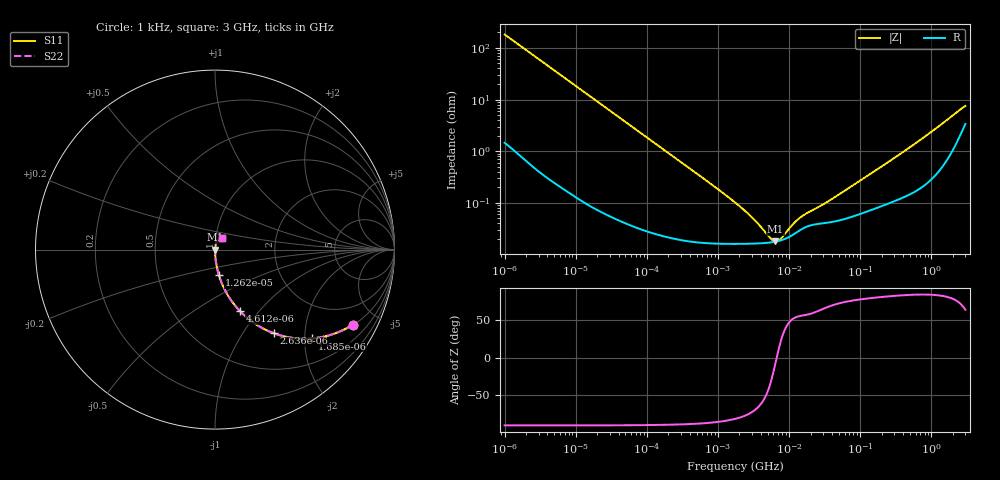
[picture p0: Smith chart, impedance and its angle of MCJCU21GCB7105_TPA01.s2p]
! MCJCU21GCB7105_TPA01  S-PARAMETER MODEL  ( Standard Model )
! Model Generated by TAIYO YUDEN Corporation (http://www.ty-top.com)
! Version 1.0
! TAIYO YUDEN Control No. 220601
! Copyright(c) 2015 TAIYO YUDEN CO.,LTD. All Rights Reserved.
! Product Description (link to TY-COMPAS)
! https://ds.yuden.co.jp/TYCOMPAS/or/detail?pn=MCJCU21GCB7105KTPA01&u=M
! Products Name : Multilayer Ceramic Capacitors
! Characteristics :
!  Capacitance : 1 [uF] , Rated Voltage : 50 [V] , TCC : X7R
!  Case Size : 2.0 x 1.25 / 0.079 x 0.049 [mm/inch] , Thickness : 1.25 / 0.049 [mm/inch]
!  (Conditions: Temperature = 25 [degC] , DC Bias Voltage = 0 [V])
! External Node Assignments :
!  1  o---| |---o  2
! GND o---------o GND
! Frequency Range : 1kHz  -  3GHz  [ 401 STEP ]
# MHZ S RI R 50
! Freq[MHz].  S11 Real  S11 Imag  S21 Real  S21 Imag  S12 Real  S12 Imag  S22 Real  S22 Imag
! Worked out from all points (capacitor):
!   401 points, 1 kHz to 3 GHz, reference 50 ohm
!   read as one part in series: C = 872 nF near 1.077 kHz
!   lowest |Z| = 17.9 mohm at 6.387 MHz (marker M1)
!   series resonance near 6.679 MHz, so ESL is about 650 pH
!   S11 on the Smith chart (normalised r, x): 1 kHz: 1.03, -3.64; 1.685 kHz: 1.02, -2.17; 2.636 kHz: 1.01, -1.39; 4.612 kHz: 1.01, -0.80; 12.62 kHz: 1.00, -0.29; 3 GHz: 1.07, +0.13
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0.001  0.7666 -0.419  0.2334 0.419  0.2334 0.419  0.7666 -0.419
0.001685  0.54 -0.4947  0.46 0.4947  0.46 0.4947  0.54 -0.4947
0.002636  0.3264 -0.4655  0.6736 0.4655  0.6736 0.4655  0.3264 -0.4655
0.004612  0.1382 -0.3418  0.8618 0.3418  0.8618 0.3418  0.1382 -0.3418
0.007215  0.0623 -0.2384  0.9377 0.2384  0.9377 0.2384  0.0623 -0.2384
0.01216  0.0234 -0.1477  0.9766 0.1477  0.9766 0.1477  0.0234 -0.1477
0.012621  0.0218 -0.1425  0.9782 0.1425  0.9782 0.1425  0.0218 -0.1425
0.03454  0.00335 -0.0533  0.9966 0.0533  0.9966 0.0533  0.00335 -0.0533
0.147855  0.000396 -0.0126  0.9996 0.0126  0.9996 0.0126  0.000396 -0.0126
1.732051  0.000162 -0.00101  0.9998 0.00101  0.9998 0.00101  0.000162 -0.00101
3.14518  0.000163 -0.000464  0.9998 0.000464  0.9998 0.000464  0.000163 -0.000464
5.502215  0.000172 -0.00011  0.9998 0.00011  0.9998 0.00011  0.000172 -0.00011
6.387174  0.000177 -2.53e-05  0.9998 2.53e-05  0.9998 2.53e-05  0.000177 -2.53e-05
7.696136  0.000189 8.05e-05  0.9998 -8.05e-05  0.9998 -8.05e-05  0.000189 8.05e-05
10.76485  0.000232 0.000274  0.9998 -0.000274  0.9998 -0.000274  0.000232 0.000274
13.46371  0.000283 0.000397  0.9997 -0.000397  0.9997 -0.000397  0.000283 0.000397
21.06097  0.000374 0.000613  0.9996 -0.000613  0.9996 -0.000613  0.000374 0.000613
39.69685  0.000427 0.0011  0.9996 -0.0011  0.9996 -0.0011  0.000427 0.0011
256.0921  0.00102 0.00629  0.999 -0.00629  0.999 -0.00629  0.00102 0.00629
1533.384  0.00706 0.0363  0.9929 -0.0363  0.9929 -0.0363  0.00706 0.0363
2489.759  0.0223 0.0577  0.9777 -0.0577  0.9777 -0.0577  0.0223 0.0577
3000  0.0367 0.0626  0.9633 -0.0626  0.9633 -0.0626  0.0367 0.0626
